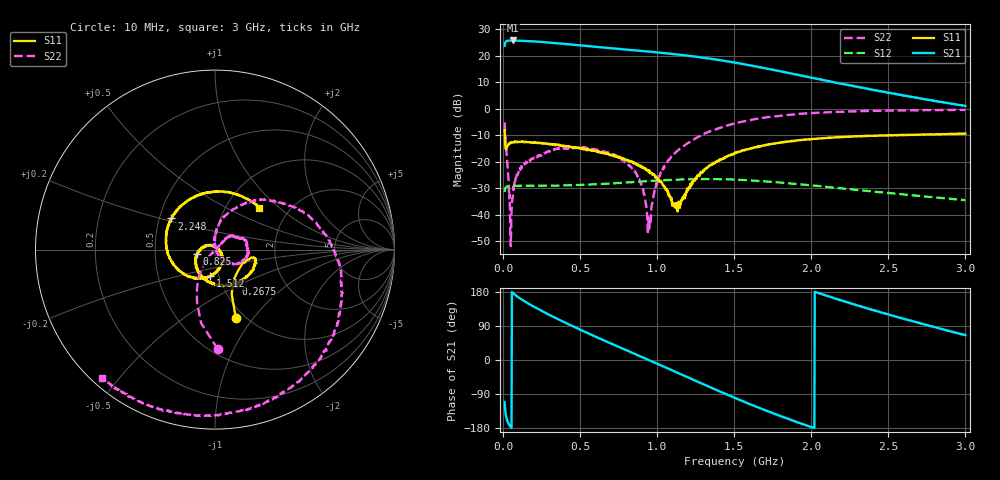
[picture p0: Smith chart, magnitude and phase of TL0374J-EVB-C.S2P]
!Agilent Technologies,E5071C,MY46523237,B.13.01
!Date: Wed Dec 15 15:57:49 2021
!Data & Calibration Information:
!Freq	S11:SOLT2(ON)	S21:SOLT2(ON)	S12:SOLT2(ON)	S22:SOLT2(ON)
!PortZ  Port1:50+j0  Port2:50+j0
!Above PortZ is port z conversion or system Z0 setting when saving the data.
!When reading, reference impedance value at option line is always used.
# Hz S dB R 50
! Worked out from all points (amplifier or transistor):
!   1197 points, 10 MHz to 3 GHz, reference 50 ohm
!   highest |S21| = 25.7 dB at 62.5 MHz (marker M1)
!   |S21| within 3 dB of that: start of sweep to 714 MHz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
!   unconditionally stable (mu >= 1): start of sweep to end of sweep
!   at 507.5 MHz: K = 1.13, MAG = 24.1 dB, |S12| = -28.7 dB
!   at 1.505 GHz: K = 1.27, MAG = 18.9 dB, |S12| = -26.7 dB
!   at 3 GHz: K = 2.17, MAG = 11.6 dB, |S12| = -34.4 dB
!   S11 on the Smith chart (normalised r, x): 10 MHz: 0.91, -0.82; 267.5 MHz: 1.16, -0.47; 825 MHz: 0.82, -0.04; 1.512 GHz: 0.91, -0.28; 2.248 GHz: 0.58, +0.22; 3 GHz: 1.42, +0.75
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1e7  -7.97 -73.1  23.72 -111.0  -31.36 78.1  -5.12 -88.5
3e7  -13.83 -13.3  25.64 -163.3  -29.25 23.6  -22.73 -128.3
4.25e7  -13.15 -11.6  25.68 -172.9  -29.12 14.7  -32.30 -131.3
6.25e7  -12.62 -14.6  25.75 177.5  -29.07 7.2  -33.70 43.6
1.525e8  -12.62 -34.1  25.51 151.7  -29.03 -7.8  -20.07 45.0
2.675e8  -12.99 -58.7  25.10 126.0  -29.00 -19.6  -16.66 28.8
3.85e8  -13.94 -81.7  24.50 101.9  -28.89 -29.9  -15.00 11.9
5.1e8  -15.10 -105.6  23.84 78.2  -28.69 -40.7  -14.77 -8.3
6.75e8  -16.82 -137.2  22.92 48.0  -28.23 -55.2  -16.39 -31.3
8.25e8  -19.70 -167.4  22.18 21.4  -27.69 -69.7  -21.82 -48.7
9.475e8  -23.62 166.9  21.52 -0.4  -27.26 -82.8  -45.19 33.4
1.0075e9  -26.98 148.3  21.18 -11.3  -27.05 -89.6  -26.31 92.8
1.1325e9  -38.71 43.6  20.43 -33.7  -26.71 -104.7  -15.78 79.3
1.2525e9  -26.01 -38.9  19.62 -55.4  -26.50 -120.0  -11.14 60.4
1.3725e9  -20.42 -67.9  18.62 -77.3  -26.48 -135.7  -7.91 42.9
1.505e9  -16.56 -97.8  17.37 -100.1  -26.70 -153.1  -5.44 23.1
1.5125e9  -16.39 -100.3  17.27 -101.4  -26.74 -154.3  -5.38 22.4
1.7325e9  -13.41 -137.6  14.91 -137.8  -27.51 178.0  -3.05 -8.0
2.005e9  -11.45 179.7  11.67 -177.9  -28.87 146.6  -1.64 -41.6
2.2475e9  -10.49 144.5  8.85 150.6  -30.29 121.5  -1.01 -67.7
2.5025e9  -10.01 110.1  5.97 120.1  -31.74 97.2  -0.67 -91.4
3e9  -9.39 43.7  1.07 65.7  -34.41 54.2  -0.41 -131.4
